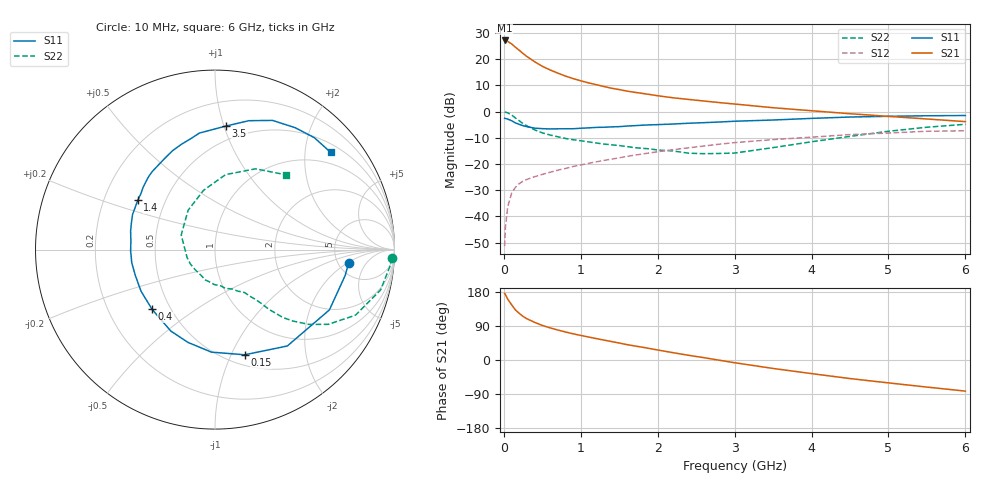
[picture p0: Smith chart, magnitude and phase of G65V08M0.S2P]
! SIEMENS Small Signal Semiconductors
! BFG193
! Si NPN RF Bipolar Junction Transistor in SOT223
! VCE = 5 V  IC = 8 mA
! Common Emitter S-Parameters:  August  1996
# GHz  S  MA  R  50
!  f  S11  S21  S12  S22
! GHz  MAG  ANG  MAG  ANG  MAG  ANG  MAG  ANG
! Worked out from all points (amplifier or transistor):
!   36 points, 10 MHz to 6 GHz, reference 50 ohm
!   highest |S21| = 27.2 dB at 10 MHz (marker M1)
!   |S21| within 3 dB of that: start of sweep to 168.1 MHz
!   unconditionally stable (mu >= 1): 965.5 MHz to 2.51 GHz
!   at 250 MHz: K = 0.46, MSG = 24.4 dB, |S12| = -26.5 dB
!   at 1.4 GHz: K = 1.07, MAG = 11.9 dB, |S12| = -18.1 dB
!   at 6 GHz: K = 0.86, MSG = 1.8 dB, |S12| = -7.3 dB
!   S11 on the Smith chart (normalised r, x): 10 MHz: 6.16, -2.15; 150 MHz: 0.61, -1.13; 400 MHz: 0.40, -0.34; 1.4 GHz: 0.35, +0.26; 3.5 GHz: 0.39, +1.02; 6 GHz: 0.69, +2.58
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0.01  0.7478 -5.9  22.82 175.8  0.0027 90.0  0.9855 -2.7
0.02  0.7393 -11.3  22.58 173.0  0.0061 87.9  0.9785 -5.6
0.05  0.7206 -27.8  21.86 160.8  0.0152 76.5  0.9496 -13.7
0.1  0.6714 -53.1  19.66 146.1  0.0275 67.2  0.864 -25.0
0.15  0.609 -74.2  16.96 132.3  0.0358 58.1  0.7564 -33.4
0.2  0.5716 -92.0  14.83 123.1  0.0422 54.4  0.6696 -38.5
0.25  0.5384 -106.3  12.84 115.0  0.0471 50.5  0.5894 -42.5
0.3  0.5162 -118.5  11.26 108.8  0.0508 49.0  0.5349 -45.0
0.4  0.4835 -136.5  8.961 99.4  0.0572 47.2  0.4485 -47.9
0.5  0.4727 -150.8  7.334 91.2  0.0633 46.4  0.3932 -49.4
0.6  0.4667 -162.1  6.254 84.9  0.0695 47.2  0.3576 -50.9
0.7  0.4695 -171.0  5.435 79.2  0.0761 47.3  0.3313 -52.7
0.9  0.4711 174.0  4.275 69.2  0.0896 47.4  0.2906 -55.5
1.1  0.4889 162.3  3.54 60.7  0.1029 47.1  0.2646 -61.1
1.4  0.5107 147.4  2.794 48.7  0.1239 45.0  0.2322 -69.9
1.7  0.539 135.7  2.336 37.1  0.1473 42.0  0.2049 -80.8
2.2  0.5794 119.1  1.835 19.3  0.1876 34.3  0.1775 -107.4
2.8  0.633 102.2  1.487 -0.5  0.2389 23.5  0.1589 -150.0
3.5  0.6912 84.9  1.186 -22.3  0.2923 7.9  0.2053 156.5
4.5  0.7879 66.0  0.911 -49.0  0.3642 -12.0  0.3365 100.9
5.5  0.8337 48.4  0.723 -71.5  0.422 -36.9  0.5033 63.4
6  0.8421 40.0  0.644 -82.1  0.4298 -51.3  0.5732 46.7
